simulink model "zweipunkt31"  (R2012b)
settings: Solver=ode45  StartTime=0.0  StopTime=50.0  RelTol=1e-3
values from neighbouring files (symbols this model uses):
  hy = 0.01    [fuellstnd_3.m]    (also in fuellstnd_31.m; regulator_1.m = 2; zweipunkt_1.m = 20; zweipunkt_2.m = 0)
  Kp = 10    [zweipunkt_1.m]    (also in zweipunkt_2.m; zweipunkt_21.m; zweipunkt_31.m; zweipunkt_32.m = 1)
  nenner_rueck = nenner_rueck{:}    [fuellstnd_3.m]    (also in fuellstnd_31.m; zweipunkt_31.m; zweipunkt_32.m)
  T1 = 1    [PID_windup1.m]    (also in pol_1.m = -5; pol_2.m = -5; pol_3.m = -5; sprung.m = x(2))
  T2 = 5    [PID_windup1.m]    (also in pol_1.m = 10; pol_2.m = 10; pol_3.m = 10; sprung.m = x(3))
  T3 = 10    [PID_windup1.m]    (also in sprung.m = x(4); sprung_1.m = x(4); zweipunkt_21.m = 20; zweipunkt_31.m = 100)
  Ts = 0.001    [fuellstnd_3.m]    (also in fuellstnd_31.m; kalman_d1.m = 0.05; kalman_d2.m = 0.1; kalman_d3.m = 0.1)
  ysoll = y.signals.values(:,2)    [ohne_kalman_1.m]    (also in zweipunkt_1.m = 500; zweipunkt_2.m = 500; zweipunkt_21.m = 500; zweipunkt_31.m = 500)
  zaehl_rueck = zaehl_rueck{:}    [fuellstnd_3.m]    (also in fuellstnd_31.m; zweipunkt_31.m; zweipunkt_32.m)

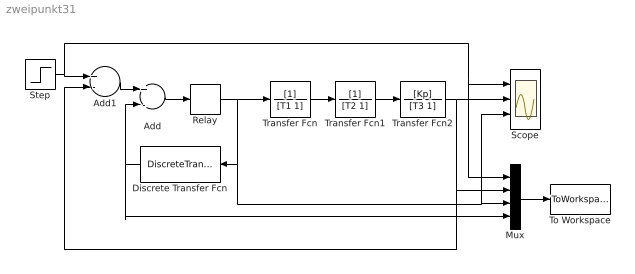
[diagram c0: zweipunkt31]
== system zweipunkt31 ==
  Add : Sum  Inputs=+-
  Add1 : Sum  Inputs=+-
  Discrete Transfer Fcn : DiscreteTransferFcn  Numerator=[zaehl_rueck]  Denominator=[nenner_rueck]  SampleTime=Ts
  Mux : Mux
  Relay : Relay  OnSwitchValue=hy  OffSwitchValue=-hy  OnOutputValue=Ustell  ZeroCross=off
  Scope : Scope  NumInputPorts=3
  Step : Step  Time=10  After=ysoll  SampleTime=0
  To Workspace : ToWorkspace  VariableName=y  SampleTime=-1  SaveFormat=Structure With Time
  Transfer Fcn : TransferFcn  Denominator=[T1 1]
  Transfer Fcn1 : TransferFcn  Denominator=[T2 1]
  Transfer Fcn2 : TransferFcn  Numerator=[Kp]  Denominator=[T3 1]
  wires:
  Transfer Fcn/1 -> Transfer Fcn1/1
  Transfer Fcn1/1 -> Transfer Fcn2/1
  Step/1 -> Mux/1, Scope/1, Add1/1
  Add/1 -> Relay/1
  Transfer Fcn2/1 -> Scope/2, Add1/2, Mux/2
  Add1/1 -> Add/1
  Relay/1 -> Transfer Fcn/1, Scope/3, Mux/3, Discrete Transfer Fcn/1
  Discrete Transfer Fcn/1 -> Add/2, Mux/4
  Mux/1 -> To Workspace/1
